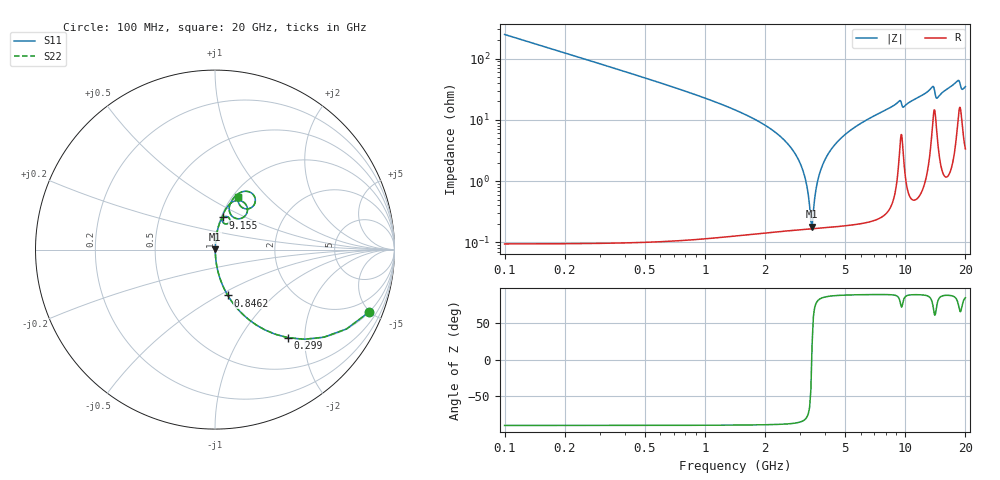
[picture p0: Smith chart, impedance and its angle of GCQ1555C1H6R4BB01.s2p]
!Murata Part Number: GCQ1555C1H6R4BB01
!These Parameters are Measured in Series Mode Connection
!Data Generated on Jan 08, 2026
!  o--ll--o
!Port1  Port2
!  o------o
!Operation Temp=25[degC], DC Bias Voltage=0[V]
!Freq. Start=100[MHz] Stop=20[GHz] 401[Steps]
# Hz S RI R 50
!Freq.(Hz) S11(Real) S11(Imag) S21(Real) S21(Imag) S12(Real) S12(Imag) S22(Real) S22(Imag)
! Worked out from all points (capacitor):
!   401 points, 100 MHz to 20 GHz, reference 50 ohm
!   read as one part in series: C = 6.4 pF near 199.5 MHz
!   lowest |Z| = 179 mohm at 3.433 GHz (marker M1)
!   series resonance near 3.418 GHz, so ESL is about 340 pH
!   S11 on the Smith chart (normalised r, x): 100 MHz: 1.00, -4.97; 299 MHz: 1.00, -1.65; 846.2 MHz: 1.00, -0.55; 9.155 GHz: 1.02, +0.38; 20 GHz: 1.07, +0.70
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1e8  0.8605 -0.3463  0.1395 0.3463  0.1395 0.3463  0.8605 -0.3463
2.99e8  0.4052 -0.4904  0.5948 0.4904  0.5948 0.4904  0.4052 -0.4904
4.98e8  0.1932 -0.3938  0.8068 0.3938  0.8068 0.3938  0.1932 -0.3938
8.4625e8  0.0715 -0.2557  0.9285 0.2557  0.9285 0.2557  0.0715 -0.2557
2.73675e9  0.00261 -0.0325  0.9974 0.0325  0.9974 0.0325  0.00261 -0.0325
3.085e9  0.00183 -0.0149  0.9982 0.0149  0.9982 0.0149  0.00183 -0.0149
3.23425e9  0.0017 -0.00801  0.9983 0.00801  0.9983 0.00801  0.0017 -0.00801
3.33375e9  0.00166 -0.00361  0.9983 0.00361  0.9983 0.00361  0.00166 -0.00361
3.43325e9  0.00166 0.000662  0.9983 -0.000662  0.9983 -0.000662  0.00166 0.000662
3.7815e9  0.00192 0.0147  0.9981 -0.0147  0.9981 -0.0147  0.00192 0.0147
4.279e9  0.00285 0.033  0.9971 -0.033  0.9971 -0.033  0.00285 0.033
5.22425e9  0.00596 0.0636  0.994 -0.0636  0.994 -0.0636  0.00596 0.0636
6.7665e9  0.014 0.1078  0.986 -0.1078  0.986 -0.1078  0.014 0.1078
9.1545e9  0.0453 0.1793  0.9547 -0.1793  0.9547 -0.1793  0.0453 0.1793
1.005e10  0.0393 0.1648  0.9607 -0.1648  0.9607 -0.1648  0.0393 0.1648
1.338325e10  0.1163 0.2724  0.8837 -0.2724  0.8837 -0.2724  0.1163 0.2724
1.3831e10  0.1758 0.2448  0.8242 -0.2448  0.8242 -0.2448  0.1758 0.2448
1.437825e10  0.0995 0.1824  0.9005 -0.1824  0.9005 -0.1824  0.0995 0.1824
1.67165e10  0.1137 0.298  0.8863 -0.298  0.8863 -0.298  0.1137 0.298
1.8607e10  0.2248 0.2764  0.7752 -0.2764  0.7752 -0.2764  0.2248 0.2764
1.915425e10  0.1583 0.2307  0.8417 -0.2307  0.8417 -0.2307  0.1583 0.2307
2e10  0.1308 0.2925  0.8692 -0.2925  0.8692 -0.2925  0.1308 0.2925
